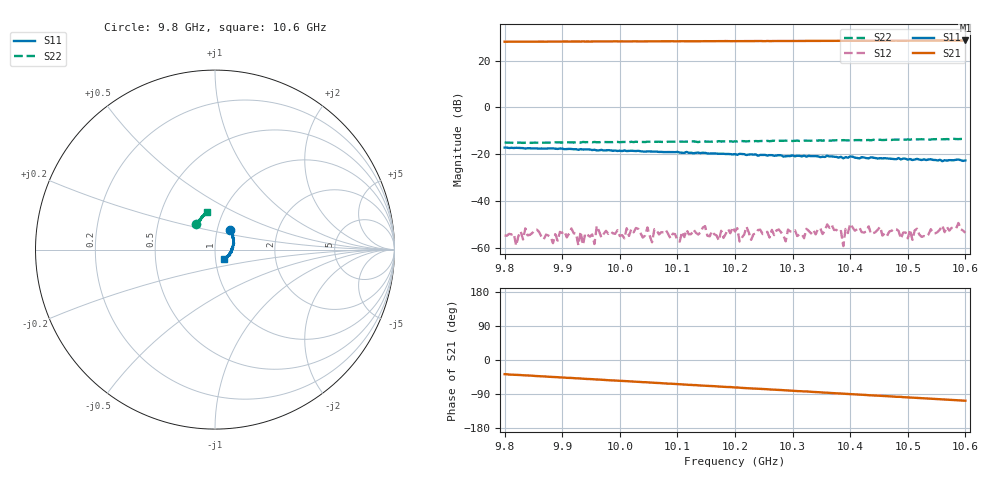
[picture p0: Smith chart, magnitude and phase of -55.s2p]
!Agilent Technologies,E8361C,US49010292,A.09.42.06
!Agilent E8361C: A.09.42.06
!Date: Tuesday, October 15, 2024 21:48:52
!Correction: S11(Full 2 Port(1,2))
!S21(Full 2 Port(1,2))
!S12(Full 2 Port(1,2))
!S22(Full 2 Port(1,2))
!S2P File: Measurements: S11, S21, S12, S22:
# Hz S  dB  R 50
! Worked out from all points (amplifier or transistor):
!   201 points, 9.8 GHz to 10.6 GHz, reference 50 ohm
!   highest |S21| = 28.6 dB at 10.6 GHz (marker M1)
!   |S21| within 3 dB of that: start of sweep to end of sweep
!   unconditionally stable (mu >= 1): start of sweep to end of sweep
!   at 9.932 GHz: K = 8.51, MAG = 28.3 dB, |S12| = -53.1 dB
!   at 10.2 GHz: K = 8.25, MAG = 28.5 dB, |S12| = -53.0 dB
!   at 10.6 GHz: K = 8.47, MAG = 28.8 dB, |S12| = -53.6 dB
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9.8e9  -17.18 51.9  28.04 -37.4  -54.67 57.3  -15.03 126.5
9.82e9  -17.25 49.5  28.09 -39.2  -59.00 70.7  -15.04 126.4
9.856e9  -17.52 45.2  28.09 -42.4  -52.21 52.8  -15.06 123.5
9.884e9  -17.50 42.1  28.09 -44.8  -58.01 26.8  -15.01 123.5
9.916e9  -17.76 40.2  28.13 -47.4  -51.70 40.1  -14.95 122.5
9.936e9  -17.98 39.0  28.20 -49.5  -58.71 78.6  -14.76 121.8
9.94e9  -17.93 37.4  28.12 -49.9  -53.83 48.5  -14.84 121.7
9.956e9  -18.10 37.0  28.16 -51.0  -58.35 40.9  -14.76 121.7
9.96e9  -18.38 35.3  28.17 -51.5  -50.67 51.8  -14.88 121.3
9.968e9  -18.14 35.1  28.13 -52.1  -55.56 52.0  -14.82 120.8
9.992e9  -18.44 33.0  28.22 -54.2  -53.97 44.0  -14.73 121.4
1.0068e10  -19.02 24.2  28.23 -60.7  -54.23 36.3  -14.65 119.2
1.02e10  -19.94 7.4  28.29 -72.6  -53.00 50.2  -14.50 114.6
1.0288e10  -20.85 -1.1  28.36 -80.1  -57.20 29.1  -14.18 112.4
1.0292e10  -20.77 -3.4  28.36 -80.5  -52.17 29.3  -14.31 113.1
1.0336e10  -20.82 -9.0  28.37 -84.3  -52.34 23.1  -14.14 111.2
1.0368e10  -20.91 -11.3  28.40 -87.2  -50.18 34.6  -14.14 109.9
1.0384e10  -21.11 -17.2  28.40 -88.6  -52.78 17.0  -14.12 109.8
1.0388e10  -21.75 -15.4  28.38 -89.0  -59.26 36.4  -13.98 109.4
1.04e10  -20.97 -20.1  28.39 -89.9  -49.74 20.7  -14.10 109.8
1.0468e10  -21.88 -29.2  28.47 -95.9  -52.98 28.6  -13.86 107.2
1.06e10  -22.66 -48.3  28.58 -107.5  -53.57 21.1  -13.43 102.7
